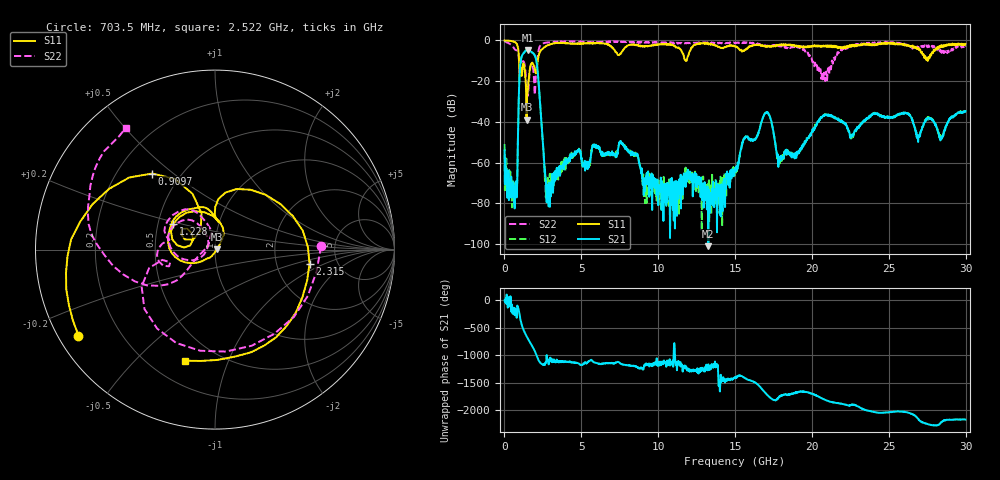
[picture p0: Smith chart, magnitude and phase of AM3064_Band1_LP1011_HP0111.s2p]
# Hz S DB R 50.0
!freq dBS11 angS11 dBS21 angS21 dBS12 angS12 dBS22 angS22
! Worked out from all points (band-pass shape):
!   1600 points, 10 MHz to 29.98 GHz, reference 50 ohm
!   highest |S21| = -4.73 dB at 1.528 GHz (marker M1); lowest = -101.0 dB at 13.26 GHz (marker M2)
!   |S21| within 3 dB of the highest: 1.128 GHz to 1.994 GHz (865.5 MHz wide, 55.4 % of centre)
!   lowest |S11| = -38.9 dB at 1.435 GHz (marker M3), VSWR 1.02, Z = 51.1 + j0.21 ohm
!   |S11| at or under -10 dB: 949.6 MHz to 2.163 GHz (1.213 GHz wide, 78 % of centre); 11.8054 GHz to 11.84035 GHz (34.95 MHz wide, 0.296 % of centre)
!   |S22| runs from -27.2 to -0.3 dB; largest |S21 - S12| = 0.0075
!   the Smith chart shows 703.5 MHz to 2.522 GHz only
!   S11 on the Smith chart (normalised r, x): 703.5 MHz: 0.06, -0.29; 909.7 MHz: 0.35, +0.42; 1.228 GHz: 0.60, +0.19; 2.315 GHz: 3.11, -0.68; 2.522 GHz: 0.34, -0.71
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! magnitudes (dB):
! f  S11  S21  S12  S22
! 10 MHz  0.0  -54.1  -50.9  -0.3
! 703.5 MHz  -0.9  -75.7  -70.0  -4.6
! 909.7 MHz  -5.2  -35.7  -35.5  -6.8
! 1.06 GHz  -13.4  -10.1  -10.1  -10.0
! 1.228 GHz  -11.3  -6.4  -6.4  -10.2
! 1.435 GHz  -38.9  -4.9  -4.8  -20.2
! 1.528 GHz  -23.7  -4.7  -4.7  -27.2
! 2.016 GHz  -15.8  -8.2  -8.1  -20.8
! 2.315 GHz  -5.5  -30.8  -30.6  -2.7
! 2.522 GHz  -3.9  -52.7  -52.3  -1.5
! 2.878 GHz  -2.2  -81.5  -68.5  -0.9
! 5.015 GHz  -1.5  -57.7  -57.1  -0.6
! 7.62 GHz  -5.8  -50.5  -50.5  -0.7
! 10 GHz  -2.0  -80.9  -71.1  -1.0
! 13.26 GHz  -1.6  -101.0  -70.4  -1.0
! 15 GHz  -3.0  -62.7  -64.5  -1.3
! 17.01 GHz  -3.2  -35.4  -35.3  -2.7
! 17.93 GHz  -1.9  -58.8  -57.3  -2.4
! 19.99 GHz  -3.1  -45.1  -44.8  -9.3
! 25 GHz  -1.2  -37.7  -37.7  -1.1
! 28.41 GHz  -2.4  -48.3  -48.4  -5.0
! 29.98 GHz  -1.8  -34.7  -35.1  -3.2
